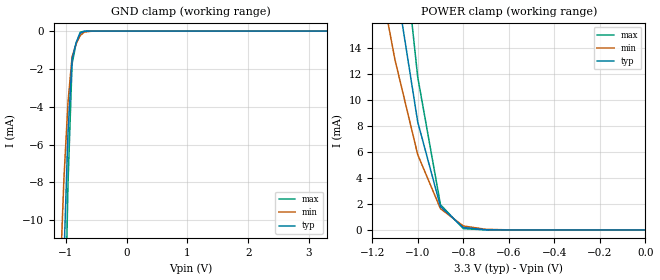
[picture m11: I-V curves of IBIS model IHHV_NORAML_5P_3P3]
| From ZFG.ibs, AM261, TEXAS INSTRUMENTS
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[Model]   IHHV_NORAML_5P_3P3
Model_type   Input
Polarity   Non-Inverting
Vinl =  0.45
Vinh =  1.35
C_comp   0.8090088p   0.6982147p   0.9645347p
|[Input load] normal
|[supplytol] 5
|[temp] ind
[Model Spec]
Vinl   0.45   0.45   0.45
Vinh   1.35   1.35   1.35
[Temperature Range]   25   125   -40
[Voltage Range]   3.3   3.135   3.465
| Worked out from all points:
|   GND clamp passes 1 mA (typ) near -0.86 V on its own axis
|   POWER clamp passes 1 mA (typ) near -0.85 V on its own axis
| Nom Voltages:
|   VDD=1.1, VDDS=3.3, VDDS18=1.8, BUS_VSSS=0, ESD_BIASFET=0, VSS=0
| Min Voltages:
|   VDD=1.045, VDDS=3.135, VDDS18=1.71, BUS_VSSS=0, ESD_BIASFET=0, VSS=0
| Max Voltages:
|   VDD=1.16, VDDS=3.465, VDDS18=1.89, BUS_VSSS=0, ESD_BIASFET=0, VSS=0
[POWER_clamp]
|   voltage   I(typ)   I(min)   I(max)
-3.3V     371.2mA    388mA      505mA
-1.133V   23.9mA     16.18mA    34.49mA
-1.1V     19.44mA    13.09mA    28.17mA
-1.067V   15.73mA    10.66mA    22.7mA
-1.033V   12.01mA    8.222mA    17.23mA
-1V       8.302mA    5.786mA    11.76mA
-900mV    1.797mA    1.632mA    1.94mA
-800mV    189uA      307.3uA    103.9uA
-700mV    15.91uA    49.24uA    4.314uA
-600mV    1.307uA    7.612uA    187.5nA
0V        882.7pA    2.251nA    3.101nA
[GND_clamp]
|   voltage   I(typ)   I(min)   I(max)
-3.3V     -581.8mA   -520.5mA   -861.2mA
-1.1V     -21.15mA   -13.37mA   -33.16mA
-1.033V   -11.94mA   -7.783mA   -18.55mA
-966.7mV  -5.39mA    -3.782mA   -8.085mA
-900mV    -1.486mA   -1.371mA   -1.752mA
-833.3mV  -616.2uA   -677.5uA   -645.7uA
-766.7mV  -124.3uA   -239.5uA   -62.57uA
-700mV    -10.21uA   -56.79uA   -2.083uA
-500mV    -38.4nA    -763.8nA   -4.996nA
3.3V      0A         0A         0A
